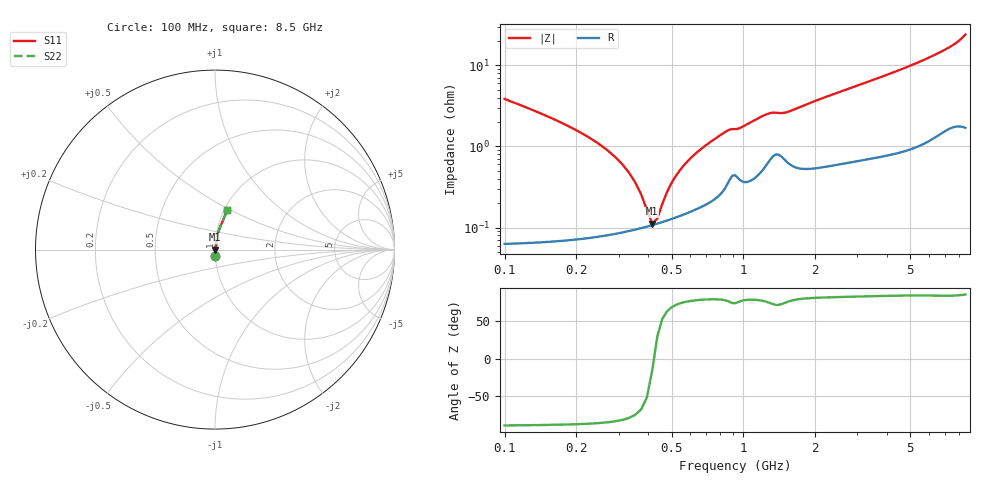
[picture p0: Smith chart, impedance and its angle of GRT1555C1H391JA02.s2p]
!Murata Part Number: GRT1555C1H391JA02
!These Parameters are Measured in Series Mode Connection
!Data Generated on Jun 19, 2026
!  o--ll--o
!Port1  Port2
!  o------o
!Operation Temp=25[degC], DC Bias Voltage=0[V]
!Freq. Start=100[MHz] Stop=9[GHz] 401[Steps]
# Hz S RI R 50
!Freq.(Hz) S11(Real) S11(Imag) S21(Real) S21(Imag) S12(Real) S12(Imag) S22(Real) S22(Imag)
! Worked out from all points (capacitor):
!   401 points, 100 MHz to 8.5 GHz, reference 50 ohm
!   read as one part in series: C = 390 pF near 142 MHz
!   lowest |Z| = 111 mohm at 415 MHz (marker M1)
!   series resonance near 421.7 MHz, so ESL is about 360 pH
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1e8  0.00211 -0.0384  0.9979 0.0384  0.9979 0.0384  0.00211 -0.0384
1.42e8  0.0013 -0.0254  0.9987 0.0254  0.9987 0.0254  0.0013 -0.0254
2.89e8  0.000888 -0.00746  0.9991 0.00746  0.9991 0.00746  0.000888 -0.00746
3.31e8  0.000925 -0.00471  0.9991 0.00471  0.9991 0.00471  0.000925 -0.00471
3.73e8  0.000988 -0.00237  0.999 0.00237  0.999 0.00237  0.000988 -0.00237
3.94e8  0.00103 -0.00131  0.999 0.00131  0.999 0.00131  0.00103 -0.00131
4.15e8  0.00107 -0.000305  0.9989 0.000305  0.9989 0.000305  0.00107 -0.000305
4.36e8  0.00112 0.000645  0.9989 -0.000645  0.9989 -0.000645  0.00112 0.000645
4.57e8  0.00117 0.00155  0.9988 -0.00155  0.9988 -0.00155  0.00117 0.00155
5.2e8  0.00134 0.00406  0.9987 -0.00406  0.9987 -0.00406  0.00134 0.00406
5.83e8  0.00155 0.00635  0.9985 -0.00635  0.9985 -0.00635  0.00155 0.00635
6.67e8  0.00188 0.00917  0.9981 -0.00917  0.9981 -0.00917  0.00188 0.00917
7.93e8  0.00267 0.0132  0.9973 -0.0132  0.9973 -0.0132  0.00267 0.0132
8.56e8  0.00363 0.0151  0.9964 -0.0151  0.9964 -0.0151  0.00363 0.0151
1.234e9  0.00616 0.0236  0.9938 -0.0236  0.9938 -0.0236  0.00616 0.0236
1.507e9  0.0072 0.0251  0.9928 -0.0251  0.9928 -0.0251  0.0072 0.0251
2.116e9  0.00692 0.0379  0.9931 -0.0379  0.9931 -0.0379  0.00692 0.0379
2.914e9  0.00931 0.0533  0.9907 -0.0533  0.9907 -0.0533  0.00931 0.0533
4.3e9  0.0147 0.0808  0.9853 -0.0808  0.9853 -0.0808  0.0147 0.0808
5.707e9  0.0236 0.1125  0.9764 -0.1125  0.9764 -0.1125  0.0236 0.1125
7.114e9  0.0395 0.1512  0.9605 -0.1512  0.9605 -0.1512  0.0395 0.1512
8.5e9  0.0684 0.2194  0.9316 -0.2194  0.9316 -0.2194  0.0684 0.2194
